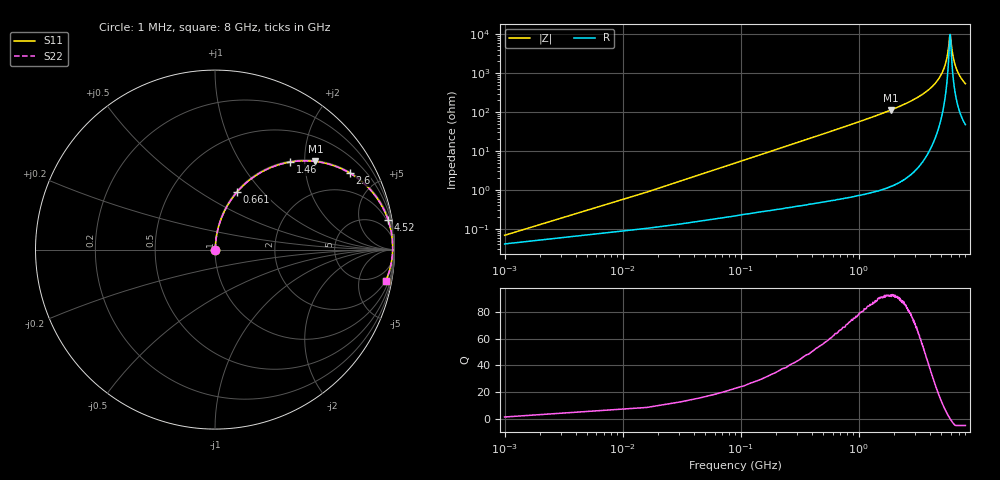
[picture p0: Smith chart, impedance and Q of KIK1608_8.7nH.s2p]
!version-2
!date-01.2022
!Series
# MHz S RI R 50
!Freq ReS11 ImS11 ReS21 ImS21 ReS12 ImS12 ReS22 ImS22
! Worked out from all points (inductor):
!   535 points, 1 MHz to 8 GHz, reference 50 ohm
!   read as one part in series: L = 8.7 nH near 31 MHz
!   highest Q = 92.4 at 1.86 GHz (marker M1), where L = 9.65 nH
!   self-resonance near 5.93 GHz
!   S11 on the Smith chart (normalised r, x): 1 MHz: 1.00, +0.00; 661 MHz: 1.01, +0.73; 1.46 GHz: 1.02, +1.69; 2.6 GHz: 1.04, +3.51; 4.52 GHz: 1, +12; 8 GHz: 2, -11
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1  0.000422 0.000546  0.9996 -0.000546  0.9996 -0.000546  0.000422 0.000546
46  0.00224 0.025  0.9978 -0.025  0.9978 -0.025  0.00224 0.025
76  0.00372 0.0413  0.9963 -0.0413  0.9963 -0.0413  0.00372 0.0413
136  0.00807 0.0736  0.9919 -0.0736  0.9919 -0.0736  0.00807 0.0736
226  0.0182 0.1211  0.9818 -0.1211  0.9818 -0.1211  0.0182 0.1211
331  0.0355 0.1744  0.9645 -0.1744  0.9645 -0.1744  0.0355 0.1744
661  0.1219 0.3195  0.8781 -0.3195  0.8781 -0.3195  0.1219 0.3195
1340  0.3732 0.4779  0.6268 -0.4779  0.6268 -0.4779  0.3732 0.4779
1460  0.4185 0.4878  0.5815 -0.4878  0.5815 -0.4878  0.4185 0.4878
1860  0.5594 0.4911  0.4406 -0.4911  0.4406 -0.4911  0.5594 0.4911
2600  0.7521 0.4257  0.2479 -0.4257  0.2479 -0.4257  0.7521 0.4257
2670  0.7673 0.4164  0.2327 -0.4164  0.2327 -0.4164  0.7673 0.4164
4010  0.9362 0.2314  0.0638 -0.2314  0.0638 -0.2314  0.9362 0.2314
4520  0.965 0.1637  0.035 -0.1637  0.035 -0.1637  0.965 0.1637
5340  0.9872 0.0641  0.0128 -0.0641  0.0128 -0.0641  0.9872 0.0641
5630  0.9896 0.0328  0.0104 -0.0328  0.0104 -0.0328  0.9896 0.0328
5880  0.9901 0.00602  0.00991 -0.00602  0.00991 -0.00602  0.9901 0.00602
5940  0.99 -9.98e-05  0.01 9.98e-05  0.01 9.98e-05  0.99 -9.98e-05
6270  0.9881 -0.0326  0.012 0.0326  0.012 0.0326  0.9881 -0.0326
6680  0.983 -0.07  0.017 0.07  0.017 0.07  0.983 -0.07
7230  0.9723 -0.1168  0.0277 0.1168  0.0277 0.1168  0.9723 -0.1168
8000  0.9519 -0.174  0.0481 0.174  0.0481 0.174  0.9519 -0.174
